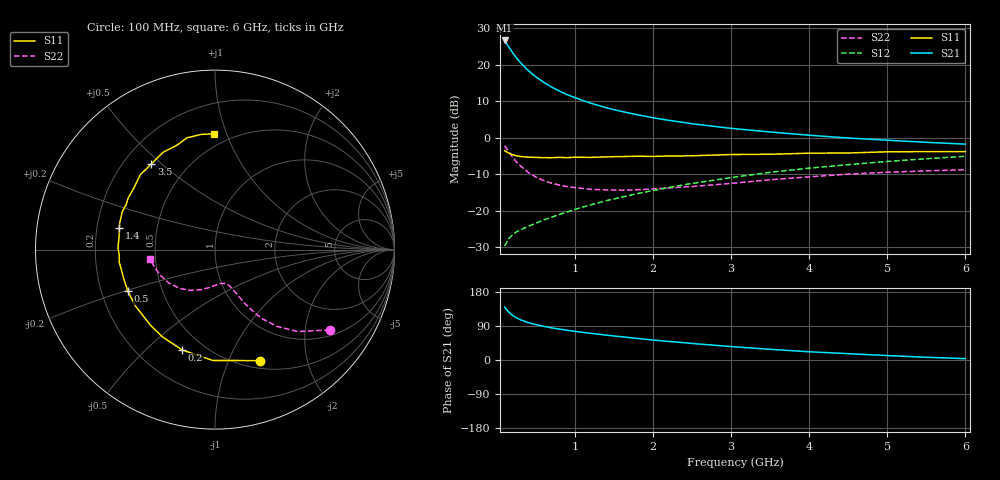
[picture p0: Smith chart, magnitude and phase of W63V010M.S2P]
! SIEMENS Small Signal Semiconductors
! BFR193W
! Si NPN RF Bipolar Junction Transistor in SOT323
! VCE = 3 V  IC = 10 mA
! Common Emitter S-Parameters:  September  1992
# GHz  S  MA  R  50
!  f  S11  S21  S12  S22
! GHz  MAG  ANG  MAG  ANG  MAG  ANG  MAG  ANG
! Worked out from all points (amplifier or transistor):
!   28 points, 100 MHz to 6 GHz, reference 50 ohm
!   highest |S21| = 26.6 dB at 100 MHz (marker M1)
!   |S21| within 3 dB of that: start of sweep to 191.5 MHz
!   unconditionally stable (mu >= 1): 1.01 GHz to 2.55 GHz
!   at 300 MHz: K = 0.56, MSG = 22.9 dB, |S12| = -25.2 dB
!   at 1.5 GHz: K = 1.05, MAG = 10.9 dB, |S12| = -16.8 dB
!   at 6 GHz: K = 0.90, MSG = 1.7 dB, |S12| = -5.1 dB
!   lowest NFmin = 1.30 dB at 450 MHz
!   S11 on the Smith chart (normalised r, x): 100 MHz: 0.59, -1.31; 200 MHz: 0.38, -0.65; 500 MHz: 0.31, -0.21; 1.4 GHz: 0.30, +0.10; 3.5 GHz: 0.31, +0.46; 6 GHz: 0.41, +0.91
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0.1  0.667 -68.0  21.47 139.7  0.0328 60.9  0.7802 -35.0
0.15  0.6178 -91.2  17.67 127.0  0.0413 54.0  0.6484 -44.8
0.2  0.5882 -108.1  14.74 117.9  0.0469 50.5  0.5477 -51.2
0.25  0.5678 -120.9  12.47 111.5  0.0513 48.9  0.4687 -55.5
0.3  0.5542 -130.4  10.76 106.4  0.0547 48.5  0.4147 -58.0
0.4  0.5431 -144.8  8.362 98.8  0.0612 49.5  0.3371 -61.3
0.5  0.5382 -154.4  6.821 93.4  0.0676 51.4  0.29 -63.1
0.6  0.534 -162.1  5.753 88.9  0.0748 53.5  0.2591 -64.9
0.7  0.5334 -167.7  4.951 85.0  0.0816 55.4  0.2391 -66.0
0.8  0.5385 -172.8  4.371 81.6  0.0889 57.1  0.2252 -67.5
0.9  0.5343 -177.0  3.9 78.5  0.0964 58.4  0.2146 -68.4
1  0.5409 179.1  3.544 75.6  0.1045 59.6  0.2081 -70.0
1.2  0.5389 172.6  2.979 70.5  0.1206 61.2  0.1969 -73.7
1.4  0.5467 167.2  2.58 65.7  0.1372 62.3  0.1933 -77.3
1.8  0.5585 158.0  2.061 56.9  0.1719 63.2  0.1943 -85.6
2.2  0.5629 149.1  1.733 49.0  0.2083 62.8  0.2048 -93.4
2.5  0.5665 143.4  1.554 43.6  0.2366 61.8  0.215 -99.3
3  0.5893 134.8  1.345 35.4  0.285 59.4  0.2374 -109.7
3.5  0.5943 126.7  1.199 28.2  0.3361 55.9  0.2659 -121.3
4.5  0.6188 110.2  0.992 16.7  0.4281 47.6  0.3178 -144.1
5.5  0.6463 96.7  0.866 7.2  0.5161 38.8  0.3521 -164.6
6  0.6452 90.4  0.818 3.6  0.5573 33.8  0.3648 -171.8
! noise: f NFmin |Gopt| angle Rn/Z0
0.45  1.3  0.22  143  0.11
0.9  1.3  0.34  160  0.11
1.8  2.05  0.54  -153  0.14
